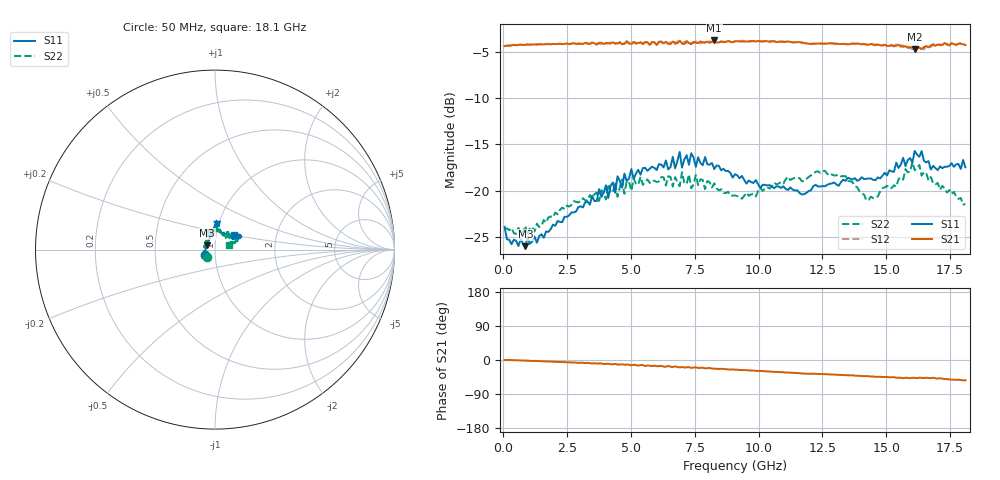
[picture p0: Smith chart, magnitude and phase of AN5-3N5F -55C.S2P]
! Network Analyzer HP8720D.06.14 Serial No. US36140669
! 27 Jun 2005  11:12:18
! Frequency  S11  S21  S12  S22
# HZ  S  DB R 50
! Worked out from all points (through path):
!   201 points, 50 MHz to 18.1 GHz, reference 50 ohm
!   highest |S21| = -3.70 dB at 8.263 GHz (marker M1); lowest = -4.7 dB at 16.11 GHz (marker M2)
!   group delay of S21, straight-line fit = 8.51 ps
!   lowest |S11| = -26.0 dB at 862.2 MHz (marker M3), VSWR 1.10, Z = 45.7 + j2.11 ohm
!   |S11| at or under -10 dB: start of sweep to end of sweep
!   |S22| runs from -24.9 to -16.9 dB; largest |S21 - S12| = 0.024
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5e7  -23.94 -148.9  -4.31 -0.1  -4.31 -0.0  -24.20 -140.1
8.6225e8  -26.04 152.6  -4.18 -1.7  -4.16 -1.5  -23.85 162.1
3.1185e9  -21.83 106.3  -4.08 -7.4  -4.10 -7.8  -20.84 121.3
4.382e9  -20.25 93.2  -4.05 -10.3  -3.98 -11.6  -19.09 110.2
4.47225e9  -18.45 88.5  -4.03 -11.9  -3.97 -10.6  -20.67 113.2
4.65275e9  -19.69 87.8  -4.12 -11.4  -3.91 -12.1  -18.81 111.0
4.743e9  -18.15 90.6  -4.05 -12.6  -4.05 -11.6  -20.35 106.6
6.09675e9  -17.13 86.3  -3.87 -16.4  -3.81 -16.1  -19.00 93.7
6.7285e9  -17.59 89.7  -3.95 -16.6  -4.12 -17.7  -18.54 85.6
6.909e9  -15.81 87.3  -3.72 -19.6  -3.87 -18.4  -19.52 83.3
6.99925e9  -17.51 86.2  -4.02 -18.5  -4.07 -20.1  -18.00 84.3
7.36025e9  -15.95 79.6  -4.12 -20.7  -3.93 -19.6  -19.77 87.0
7.54075e9  -17.43 80.2  -3.95 -19.1  -3.80 -21.1  -18.31 86.4
8.26275e9  -17.68 87.4  -3.70 -23.0  -3.85 -23.6  -19.22 71.9
9.075e9  -18.23 87.4  -3.80 -25.3  -3.78 -25.4  -20.53 63.8
1.21435e10  -19.54 62.5  -4.06 -36.0  -4.02 -36.2  -18.21 54.6
1.3407e10  -18.94 46.0  -4.09 -39.9  -4.07 -40.1  -18.43 51.4
1.421925e10  -18.72 33.5  -4.15 -42.4  -4.14 -42.6  -21.06 47.4
1.512175e10  -17.80 27.8  -4.29 -45.7  -4.16 -45.5  -19.76 39.4
1.61145e10  -15.70 28.9  -4.65 -47.0  -4.34 -47.5  -17.80 28.8
1.674625e10  -17.72 29.5  -4.24 -47.9  -4.42 -48.3  -18.53 19.2
1.81e10  -17.48 37.7  -4.19 -53.3  -4.25 -53.9  -21.46 19.4
